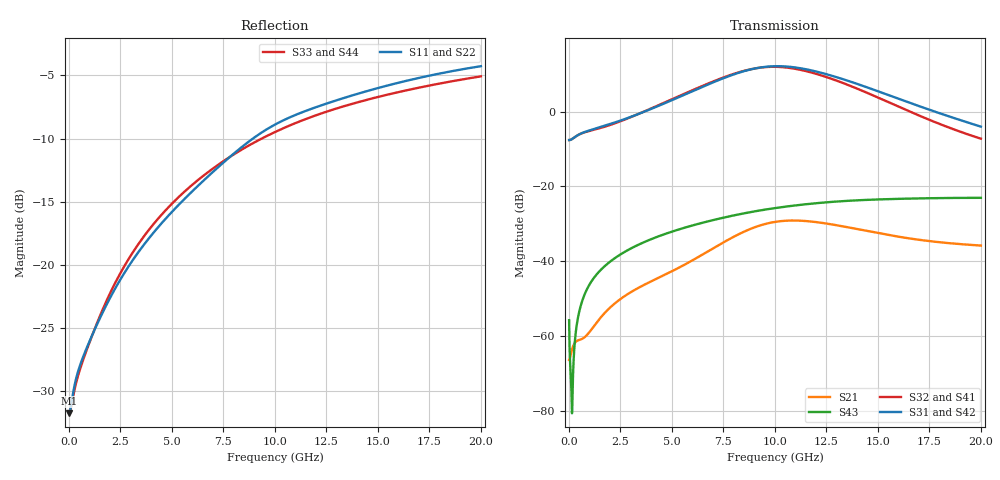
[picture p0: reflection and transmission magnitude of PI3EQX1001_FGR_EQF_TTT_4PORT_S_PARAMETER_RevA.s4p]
! NPort=4 DATA=2000 NOISE=0 GROUPDELAY=0 COMPLEX_DATAFORMAT=POLAR
! NumOfBlock=1 NumOfParam=0
! .MODEL Smodel S TSTONEFILE=PI3EQX1001_FGR_EQF_TTT_4PORT_S_PARAMETER_RevA.s4p TYPE=S
!  -- The above .MODEL line can be used for the S element in the netlist.
! The s parameter is extracted from the linear redriver, it is not bi-directional; only s(4,1)s(4,2) and s(3,1)s(3,2)
! should be the insertion loss
!Port definition:
!Port1 = input+
!Port2 = input¨C
!Port3 = output+
!Port4 = output-
# Hz S MA R  50
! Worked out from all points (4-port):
!   2000 points, 10 MHz to 20 GHz, reference 50 ohm
!   strongest paths, dB at 10 MHz, 5.01 GHz, 10.01 GHz, 15.01 GHz, 20 GHz:
!     S31: -7.6, 3.1, 12.2, 5.4, -4.0
!     S42: -7.6, 3.1, 12.1, 5.4, -4.0
!     S32: -7.6, 3.3, 12.0, 3.8, -7.2
!     S41: -7.6, 3.3, 12.0, 3.7, -7.3
!     S43: -55.8, -32.1, -25.8, -23.5, -23.1
!     S21: -66.4, -42.7, -29.5, -32.5, -35.8
!   lowest |S11| = -31.7 dB at 10 MHz (marker M1), VSWR 1.05, Z = 47.5 - j0.063 ohm
!   |S11| at or under -10 dB: start of sweep to 8.929 GHz
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1e7  0.0259 -178.5  0.0004911 2.7  3.669e-05 -0.2  4.787e-05 -0.1
     0.0004778 2.9  0.02597 -178.7  4.577e-05 -0.2  5.994e-05 -0.1
     0.417 -0.1  0.4169 179.9  0.02616 178.4  0.001615 -59.2
     0.4167 179.9  0.4168 -0.1  0.001626 -59.0  0.02612 178.4
7.03e9  0.235 -105.3  0.01434 89.0  2.189e-05 -31.0  3.209e-05 -29.7
        0.01501 87.2  0.2331 -105.3  2.903e-05 -25.8  4.026e-05 -24.9
        2.484 -55.0  2.551 129.7  0.242 -111.8  0.03565 56.7
        2.541 129.7  2.478 -54.9  0.03563 56.7  0.2419 -111.8
9.07e9  0.3223 -108.0  0.02775 62.3  1.972e-05 -27.8  3.271e-05 -32.7
        0.02875 60.8  0.3201 -108.0  3.043e-05 -25.9  3.814e-05 -24.3
        3.799 -112.5  3.8 72.1  0.3075 -114.5  0.04672 44.2
        3.781 72.2  3.792 -112.4  0.04667 44.1  0.3073 -114.5
1.087e10  0.3884 -113.3  0.03385 27.1  2.198e-05 -21.4  3.419e-05 -44.0
          0.03501 25.9  0.3855 -113.4  3.241e-05 -36.5  4.023e-05 -22.8
          3.94 -172.8  3.788 12.3  0.3607 -117.6  0.05532 32.0
          3.766 12.5  3.934 -172.8  0.05519 32.0  0.3604 -117.5
1.33e10  0.4565 -118.7  0.02819 -7.2  2.95e-05 -37.3  3.017e-05 -67.0
         0.02923 -8.2  0.4528 -118.8  2.833e-05 -57.7  4.688e-05 -34.4
         2.722 116.4  2.419 -56.7  0.4235 -121.7  0.06374 15.4
         2.403 -56.5  2.717 116.4  0.06359 15.5  0.4235 -121.7
1.582e10  0.5217 -123.3  0.02078 -22.6  2.924e-05 -70.4  2.173e-05 -97.0
          0.02167 -23.7  0.5173 -123.4  1.93e-05 -83.8  4.385e-05 -57.4
          1.552 60.5  1.229 -108.0  0.4793 -125.5  0.0681 -0.4
          1.221 -107.5  1.549 60.6  0.06802 -0.3  0.479 -125.5
2e10  0.6117 -130.6  0.01556 -27.4  1.608e-05 -147.0  1.363e-05 148.1
      0.01619 -29.5  0.6063 -130.6  9.195e-06 133.3  1.901e-05 -97.2
      0.6302 -6.5  0.4353 -156.1  0.5574 -131.1  0.07041 -23.6
      0.4339 -155.2  0.6285 -6.4  0.07037 -23.6  0.5573 -131.1
